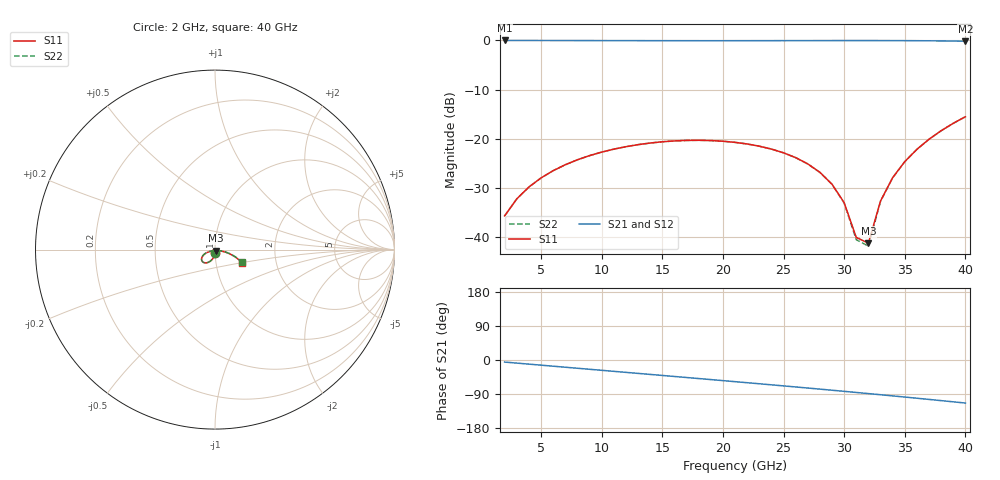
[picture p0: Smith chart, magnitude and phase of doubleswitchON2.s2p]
# GHZ S RI R 50
!Output file by Shape3_31
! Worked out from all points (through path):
!   39 points, 2 GHz to 40 GHz, reference 50 ohm
!   highest |S21| = -0.04 dB at 2 GHz (marker M1); lowest = -0.2 dB at 40 GHz (marker M2)
!   group delay of S21, straight-line fit = 7.83 ps
!   lowest |S11| = -41.1 dB at 32 GHz (marker M3), VSWR 1.02, Z = 50.7 - j0.568 ohm
!   |S11| at or under -10 dB: start of sweep to end of sweep
!   |S22| runs from -41.8 to -15.5 dB; largest |S21 - S12| = 4.2e-14
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2  0.00181 -0.0165  0.9907 -0.0947  0.9907 -0.0947  0.00181 -0.0165
3  -1.77e-05 -0.0246  0.9848 -0.1415  0.9848 -0.1415  -2.67e-05 -0.0246
5  -0.00588 -0.0397  0.9663 -0.234  0.9663 -0.234  -0.00591 -0.0397
7  -0.0142 -0.0528  0.939 -0.3242  0.939 -0.3242  -0.0143 -0.0527
9  -0.0244 -0.063  0.9033 -0.4112  0.9033 -0.4112  -0.0245 -0.063
12  -0.0414 -0.0723  0.8348 -0.5342  0.8348 -0.5342  -0.0415 -0.0722
15  -0.0576 -0.0735  0.7499 -0.6462  0.7499 -0.6462  -0.0578 -0.0734
18  -0.0698 -0.0669  0.65 -0.7458  0.65 -0.7458  -0.0701 -0.0667
21  -0.0748 -0.054  0.5366 -0.8313  0.5366 -0.8313  -0.075 -0.0536
25  -0.0651 -0.0314  0.3662 -0.9206  0.3662 -0.9206  -0.0653 -0.0309
27  -0.0519 -0.0204  0.2734 -0.9531  0.2734 -0.9531  -0.0521 -0.0197
28  -0.0431 -0.0156  0.2254 -0.966  0.2254 -0.966  -0.0432 -0.0149
29  -0.0328 -0.0115  0.1763 -0.9765  0.1763 -0.9765  -0.0329 -0.0107
30  -0.021 -0.00833  0.1262 -0.9845  0.1262 -0.9845  -0.0211 -0.00747
31  -0.00779 -0.00629  0.0753 -0.9898  0.0753 -0.9898  -0.00785 -0.00537
32  0.00675 -0.0056  0.0236 -0.9923  0.0236 -0.9923  0.00673 -0.00463
33  0.0225 -0.0065  -0.0286 -0.9918  -0.0286 -0.9918  0.0225 -0.00546
34  0.0394 -0.00918  -0.0812 -0.9883  -0.0812 -0.9883  0.0395 -0.00809
35  0.0571 -0.0139  -0.134 -0.9815  -0.134 -0.9815  0.0573 -0.0127
36  0.0756 -0.0207  -0.1867 -0.9714  -0.1867 -0.9714  0.0758 -0.0195
38  0.1136 -0.0416  -0.291 -0.9408  -0.291 -0.9408  0.114 -0.0404
40  0.151 -0.0729  -0.3915 -0.8959  -0.3915 -0.8959  0.1516 -0.0716
